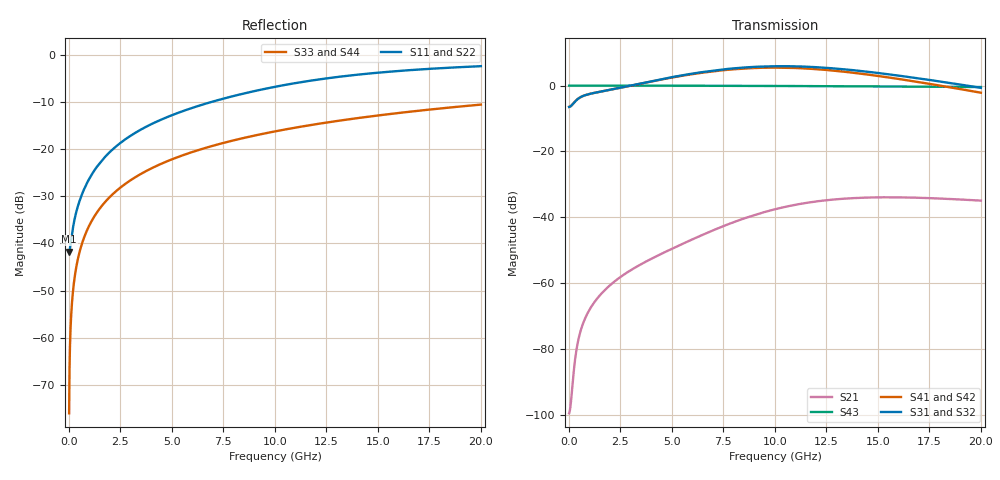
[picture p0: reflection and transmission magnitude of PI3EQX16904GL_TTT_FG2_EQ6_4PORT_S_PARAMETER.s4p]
! NPort=4 DATA=2000 NOISE=0 GROUPDELAY=0 COMPLEX_DATAFORMAT=POLAR
! NumOfBlock=1 NumOfParam=0
! .MODEL Smodel S TSTONEFILE=PI3EQX16904GL_TTT_FG2_EQ6_4PORT_S_PARAMETER.s4p TYPE=S
!  -- The above .MODEL line can be used for the S element in the netlist.
! The s parameter is extracted from the linear redriver, it is not bi-directional; only s(4,1)s(4,2) and s(3,1)s(3,2)
! should be the insertion loss
!Port definition:
!Port1 = input+
!Port2 = input-
!Port3 = output+
!Port4 = output-
# Hz S MA R  50
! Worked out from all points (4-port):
!   2000 points, 10 MHz to 20 GHz, reference 50 ohm
!   strongest paths, dB at 10 MHz, 5.01 GHz, 10.01 GHz, 15.01 GHz, 20 GHz:
!     S31: -6.5, 2.6, 5.9, 3.8, -0.7
!     S32: -6.5, 2.5, 5.8, 3.7, -0.8
!     S41: -6.5, 2.5, 5.5, 2.9, -2.2
!     S42: -6.5, 2.4, 5.3, 2.8, -2.3
!     S43: 0.0, 0.0, -0.1, -0.3, -0.4
!     S21: -99.6, -49.6, -37.6, -34.0, -34.9
!   lowest |S11| = -41.7 dB at 10 MHz (marker M1), VSWR 1.02, Z = 49.2 - j0.0603 ohm
!   |S11| at or under -10 dB: start of sweep to 6.871 GHz
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1e7  0.008182 -175.7  1.05e-05 7.8  0 0.0  0 0.0
     1.05e-05 7.8  0.008182 -175.7  0 0.0  0 0.0
     0.4744 0.7  0.4744 -179.3  0.0001571 -90.0  1 -0.0
     0.4744 -179.3  0.4744 0.7  1 -0.0  0.0001571 -90.0
3.8e8  0.02256 -119.7  0.0001024 118.3  0 0.0  0 0.0
       0.0001024 118.3  0.02256 -119.7  0 0.0  0 0.0
       0.6073 13.6  0.6072 -166.5  0.005969 -90.4  1 -0.3
       0.6072 -167.1  0.6071 12.8  1 -0.3  0.005969 -90.4
1.6e9  0.07608 -102.8  0.0007038 109.1  0 0.0  0 0.0
       0.0007034 109.1  0.07608 -102.8  0 0.0  0 0.0
       0.817 5.1  0.8173 -175.1  0.02512 -91.5  0.9997 -1.4
       0.8159 -177.7  0.8162 2.0  0.9997 -1.4  0.02512 -91.5
5.96e9  0.2742 -104.7  0.004596 101.1  0 0.0  0 0.0
        0.004561 101.4  0.2742 -104.7  0 0.0  0 0.0
        1.515 -37.8  1.495 141.7  0.09318 -95.6  0.9953 -5.3
        1.488 131.6  1.468 -48.9  0.9953 -5.3  0.09318 -95.6
9.64e9  0.4447 -111.9  0.01243 70.3  0 0.0  0 0.0
        0.01234 71.2  0.4446 -111.9  0 0.0  0 0.0
        1.959 -97.8  1.934 81.9  0.1496 -98.9  0.9878 -8.6
        1.872 65.3  1.848 -114.9  0.9878 -8.6  0.1496 -98.9
1.362e10  0.6075 -122.2  0.01944 21.1  0 0.0  0 0.0
          0.01936 22.5  0.6073 -122.2  0 0.0  0 0.0
          1.736 -166.1  1.714 13.7  0.2088 -102.5  0.9762 -12.1
          1.591 -9.2  1.571 170.6  0.9762 -12.1  0.2088 -102.5
2e10  0.7643 -136.3  0.0179 -37.2  0 0.0  0 0.0
      0.01789 -35.3  0.7643 -136.3  0 0.0  0 0.0
      0.9256 104.5  0.9128 -75.8  0.2986 -108.1  0.9506 -17.4
      0.7794 -107.4  0.7685 72.3  0.9506 -17.4  0.2986 -108.1
